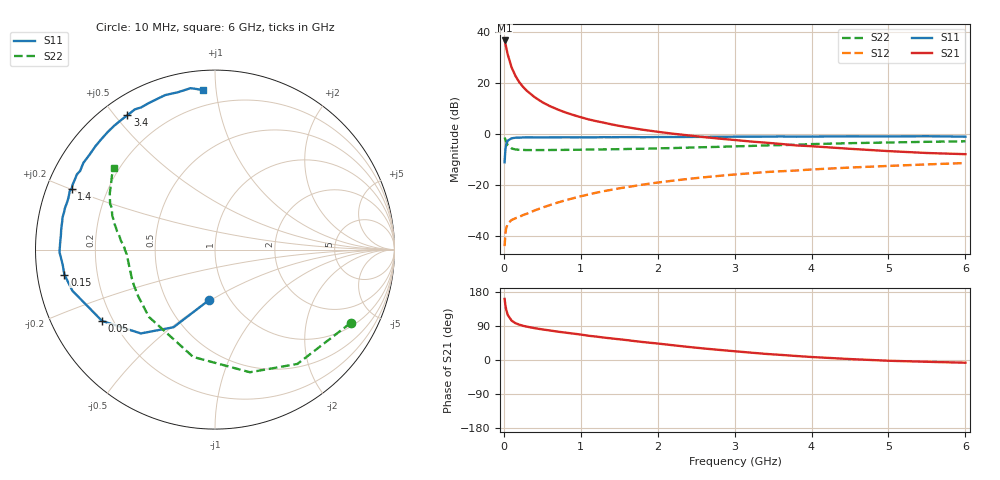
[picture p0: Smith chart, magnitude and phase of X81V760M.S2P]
! SIEMENS Small Signal Semiconductors
! BFP136W
! Si NPN RF Bipolar Junction Transistor in SOT343
! VCE = 1.75 V  IC = 60 mA
! Common Emitter S-Parameters:  September  1994
# GHz  S  MA  R  50
!  f  S11  S21  S12  S22
! GHz  MAG  ANG  MAG  ANG  MAG  ANG  MAG  ANG
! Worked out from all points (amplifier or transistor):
!   40 points, 10 MHz to 6 GHz, reference 50 ohm
!   highest |S21| = 36.7 dB at 10 MHz (marker M1)
!   |S21| within 3 dB of that: start of sweep to 32.82 MHz
!   unconditionally stable (mu >= 1): 550.6 MHz to 2.885 GHz
!   at 200 MHz: K = 0.61, MSG = 26.4 dB, |S12| = -32.4 dB
!   at 1.5 GHz: K = 1.11, MAG = 10.2 dB, |S12| = -21.2 dB
!   at 6 GHz: K = 0.98, MSG = 1.7 dB, |S12| = -11.3 dB
!   S11 on the Smith chart (normalised r, x): 10 MHz: 0.81, -0.49; 50 MHz: 0.16, -0.28; 150 MHz: 0.08, -0.08; 1.4 GHz: 0.07, +0.20; 3.4 GHz: 0.07, +0.54; 6 GHz: 0.11, +0.92
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0.01  0.281 -96.3  68.23 161.2  0.0064 70.7  0.8593 -28.4
0.02  0.4904 -118.1  59.42 145.2  0.0111 57.4  0.7853 -54.2
0.03  0.6236 -131.5  50.57 133.6  0.0143 48.8  0.7105 -74.1
0.05  0.7444 -147.7  36.53 119.2  0.0176 38.0  0.6103 -101.5
0.1  0.8268 -163.9  20.37 104.1  0.0208 33.0  0.5256 -134.4
0.15  0.8506 -170.6  13.87 97.3  0.0225 34.1  0.5009 -148.6
0.2  0.853 -174.4  10.42 93.2  0.024 36.4  0.4934 -156.3
0.25  0.8602 -177.2  8.412 90.2  0.026 39.4  0.4903 -161.1
0.3  0.8666 -179.1  7.031 88.0  0.0277 41.9  0.4874 -164.4
0.4  0.8634 177.1  5.295 84.0  0.032 46.6  0.4868 -168.7
0.5  0.8624 174.5  4.22 80.7  0.0363 50.5  0.4875 -171.5
0.6  0.8642 172.5  3.522 77.9  0.0408 53.1  0.4887 -173.4
0.7  0.8654 169.8  3.037 74.8  0.0457 55.6  0.49 -174.7
0.9  0.8664 166.4  2.377 69.7  0.0555 57.5  0.4926 -177.2
1.1  0.8651 161.9  1.946 64.0  0.0657 58.7  0.4978 -178.8
1.4  0.8681 157.0  1.552 56.9  0.0814 59.0  0.5044 178.9
2.2  0.8764 143.0  1.019 38.9  0.1226 54.7  0.5335 172.9
3.2  0.8915 126.0  0.719 19.6  0.1709 45.8  0.5864 164.0
3.4  0.8935 123.1  0.681 16.2  0.1806 43.7  0.6013 162.0
4.5  0.9046 107.9  0.516 2.5  0.2216 33.4  0.6655 151.7
5.5  0.9097 98.6  0.427 -4.7  0.2553 25.5  0.7071 144.3
6  0.8919 94.3  0.405 -7.2  0.2718 21.1  0.7231 141.2
